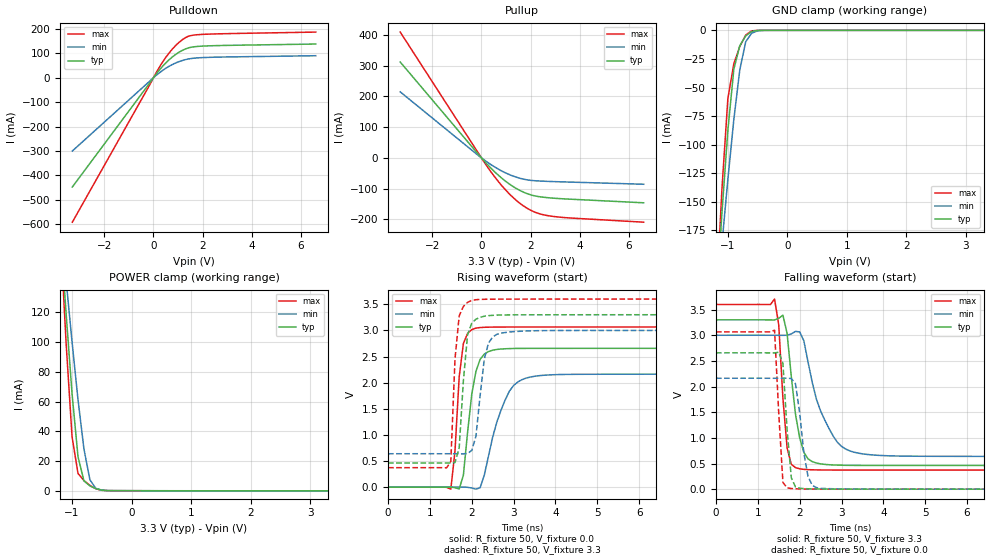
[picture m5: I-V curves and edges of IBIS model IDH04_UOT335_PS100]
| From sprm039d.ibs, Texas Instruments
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[Model]   IDH04_UOT335_PS100
| I/O with pullup
Model_type   I/O
Vinh = 2.00
Vinl = 0.80
Enable   Active-Low
Polarity   Non-Inverting
| signals   A, GZ, Y
Vmeas = 1.5
|   typ   min   max
C_comp   2.951p   2.793p   3.090p
|   typ   min   max
[Temperature Range]   25   -40   125
|   typ   min   max
[Voltage Range]   3.30V   3.00V   3.60V
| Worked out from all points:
|   slope of the pulldown table from 0 to 0.495 V, typ, clamps not added: 8.22 ohm
|   slope of the pullup table from 0 to 0.495 V, typ, clamps not added: 11.8 ohm
|   GND clamp passes 1 mA (typ) near -0.60 V on its own axis
|   POWER clamp passes 1 mA (typ) near -0.56 V on its own axis
|   rising waveform, R_fixture 50, V_fixture 0.0: 20-80 % time 242ps typ, 480ps min, 165ps max; typ from 0 V to 2.66 V
|   falling waveform, R_fixture 50, V_fixture 3.3: 20-80 % time 258ps typ, 561ps min, 160ps max; typ from 3.3 V to 0.462 V
|   rising waveform, R_fixture 50, V_fixture 3.3: 20-80 % time 158ps typ, 207ps min, 134ps max; typ from 0.462 V to 3.3 V
|   falling waveform, R_fixture 50, V_fixture 0.0: 20-80 % time 142ps typ, 201ps min, 124ps max; typ from 2.66 V to 0 V
[Pulldown]
|   Voltage   I(typ)   I(min)   I(max)
-3.3V     -448.2mA   -300.5mA   -592.5mA
200mV     26.69mA    17.06mA    36.54mA
600mV     70.53mA    44.94mA    97.01mA
800mV     87.84mA    55.83mA    121.2mA
1.1V      108.3mA    68.43mA    150.3mA
1.4V      121.9mA    76.68mA    169.3mA
1.9V      129.3mA    82.24mA    177.4mA
6.6V      138.4mA    90.43mA    187.4mA
[GND_clamp]
|   Voltage   I(typ)   I(min)   I(max)
-3.3V     -2.114A    -1.592A    -2.733A
-1.2V     -239.4mA   -245.5mA   -241.1mA
-1.1V     -159.8mA   -186.7mA   -138.7mA
-1V       -87.29mA   -130.2mA   -59.49mA
-900mV    -33.99mA   -77.9mA    -29.21mA
-800mV    -13.44mA   -34.54mA   -14.09mA
-700mV    -4.925mA   -9.943mA   -4.108mA
-600mV    -954.5uA   -2.435mA   -464.9uA
-500mV    -87.08uA   -433.5uA   -21.61uA
-400mV    -4.855uA   -53.01uA   -479.6nA
3.3V      310.9pA    4.26uA     88.82pA
[Pullup]
|   Voltage   I(typ)   I(min)   I(max)
-3.3V     311.6mA    214.5mA    409mA
-200mV    18.62mA    12.57mA    24.84mA
300mV     -26.32mA   -17.35mA   -35.69mA
900mV     -70.83mA   -45.77mA   -97.06mA
1.2V      -88.69mA   -56.59mA   -122.3mA
1.5V      -103.4mA   -64.99mA   -143.8mA
1.8V      -114.7mA   -70.84mA   -161.1mA
2.1V      -122.5mA   -74.08mA   -174.1mA
2.7V      -129.7mA   -76.64mA   -188.1mA
3.6V      -134.5mA   -78.95mA   -195.7mA
6.6V      -146.3mA   -86mA      -209.4mA
[POWER_clamp]
|   Voltage   I(typ)   I(min)   I(max)
-3.3V     1.533A     1.162A     1.984A
-1.2V     177.8mA    184.9mA    175.5mA
-1.1V     119.3mA    141.7mA    99.45mA
-1V       65.24mA    100.1mA    36.37mA
-900mV    22.87mA    61.25mA    11.62mA
-800mV    6.579mA    28.03mA    6.822mA
-700mV    3.218mA    7.342mA    3.568mA
-600mV    1.373mA    1.539mA    1.296mA
-500mV    357.3uA    353.7uA    240.6uA
-400mV    65.61uA    68.51uA    56.84uA
3.3V      -108.3uA   -68.4uA    -162.1uA
[Ramp]
|   I(typ)   I(min)   I(max)
dV/dt_r   1.594/0.234n   1.297/0.474n   1.839/0.146n
dV/dt_f   1.703/0.253n   1.417/0.558n   1.937/0.152n
[Rising Waveform]
R_fixture = 50
V_fixture = 0.0
|  pu_on
|  TIME   V(typ)   V(min)   V(max)
0s        2nV        13nV       2nV
1.5ns     546.9uV    45.16uV    -39.17mV
1.6ns     -10.74mV   233.9uV    694.5mV
1.7ns     -36.59mV   486.9uV    2.112V
1.8ns     228.2mV    580.7uV    2.748V
2ns       1.777V     -16.38mV   3.014V
2.3ns     2.547V     229.2mV    3.06V
2.8ns     2.649V     1.671V     3.064V
3.3ns     2.656V     2.087V     3.065V
10ns      2.657V     2.162V     3.066V
[Falling Waveform]
R_fixture = 50
V_fixture = 3.3
V_fixture_min = 3.0
V_fixture_max = 3.6
|  pd_on
|  TIME   V(typ)   V(min)   V(max)
0s        3.3V       3V         3.6V
1.4ns     3.298V     3V         3.705V
1.5ns     3.331V     2.999V     3.204V
1.6ns     3.392V     2.999V     1.767V
1.7ns     3.035V     3.001V     802.9mV
1.9ns     1.461V     3.075V     419.7mV
2.2ns     591.7mV    2.482V     380.4mV
2.6ns     482.6mV    1.349V     373.6mV
3.2ns     464.2mV    746mV      372.3mV
10ns      461.6mV    639mV      372mV
[Rising Waveform]
R_fixture = 50
V_fixture = 3.3
V_fixture_min = 3.0
V_fixture_max = 3.6
|  pd_off
|  TIME   V(typ)   V(min)   V(max)
0s        461.6mV    638.9mV    372mV
1.5ns     460.9mV    639.2mV    492.2mV
1.6ns     472.2mV    639.1mV    2.456V
1.7ns     751.9mV    638.2mV    3.28V
1.9ns     2.914V     643.7mV    3.537V
2ns       3.14V      703mV      3.574V
2.1ns     3.214V     971.6mV    3.588V
2.3ns     3.271V     2.451V     3.596V
2.6ns     3.292V     2.926V     3.598V
10ns      3.3V       3V         3.6V
[Falling Waveform]
R_fixture = 50
V_fixture = 0.0
|  pu_off
|  TIME   V(typ)   V(min)   V(max)
0s        2.657V     2.162V     3.066V
1.4ns     2.656V     2.162V     3.099V
1.6ns     2.449V     2.161V     131.3mV
1.7ns     1.154V     2.163V     25.5mV
1.8ns     224.7mV    2.156V     12.08mV
1.9ns     42mV       2.054V     7.412mV
2.1ns     11.07mV    702.9mV    3.087mV
2.2ns     7.764mV    246.7mV    2.236mV
2.4ns     4.18mV     30.3mV     1.297mV
10ns      301nV      10.13uV    166nV
